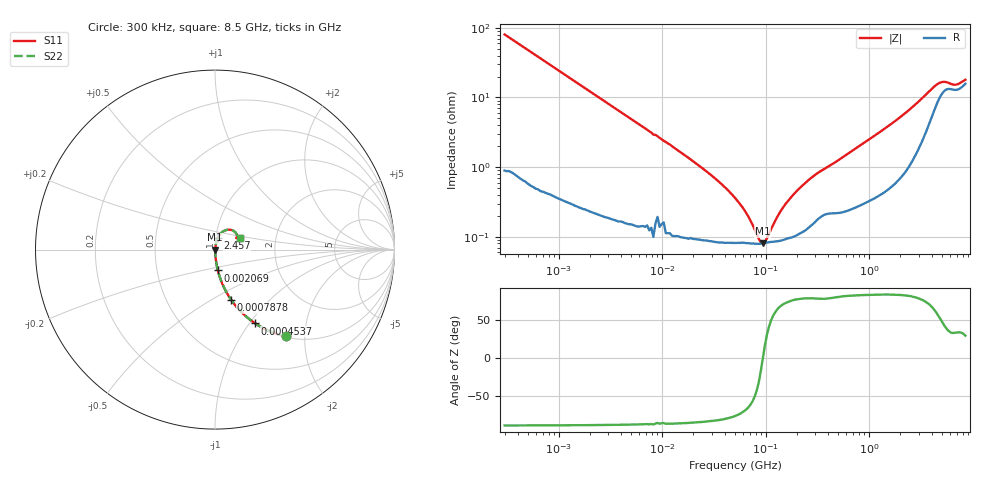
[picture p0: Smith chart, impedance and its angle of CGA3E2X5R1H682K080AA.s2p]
! S-parameter Generated by TDK Corporation
! Copyright(C) 2015 TDK Corporation.
! All Rights Reserved.
! TDK P/N: CGA3E2X5R1H682K080AA (Multilayer Ceramic Chip Capacitors)
! Property: C=6.8nF
! Size(LxWxT): 1.6x0.8x0.8mm, 0.063x0.031x0.031inches
! Model Type: s2p (Touchstone File Format Version 1.0)
! Frequency: DC=Yes Start=0.3MHz Stop=8500MHz 225points Log-sweep
! Note:
! Model Generated on Jun. 23, 2015
! Hash(MD5):
! Port Assignments:
!  1 ---| |--- 2
! Applicable Conditions:
!  Temperature = 25 degC
!  DC Bias Voltage = 0 V
!  Small Signal Operation
! Terms and conditions regarding TDK Simulation Models
! (1)This simulation model is being provided solely for informational purposes. Please refer to the specifications of the products in terms of detailed characteristics of such products.
! (2)In no event shall TDK Corporation of any of its subsidiaries be liable for any loss or damage arising, directly or indirectly,
!  From any information contained in this simulation model, including, but not limited to loss or damages arising from any inaccuracies, omissions or errors in connection with such information.
! (3)Any and all copyrights on this simulation model are owned by TDK Corporation.
!  Duplication or redistribution of this simulation model without prior written permission from TDK Corporation is prohibited.
! (4)This simulation model is subject to any modification or change without any prior notice.
! (5)Neither TDK Corporation nor any of its subsidiaries shall make any warranty, express or implied,
!  Including but not limited to the correctness, implied warranties of merchantability and fitness for a particular purpose with respect to this simulation models.
! (6)The use of this simulation model shall be deemed to have consented to the terms and conditions hereof.
# MHz S MA R 50
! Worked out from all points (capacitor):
!   224 points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, 300 kHz to 8.5 GHz, reference 50 ohm
!   read as one part in series: C = 6.59 nF near 314.1 kHz
!   lowest |Z| = 80.3 mohm at 93.93 MHz (marker M1)
!   series resonance near 94.01 MHz, so ESL is about 440 pH
!   S11 on the Smith chart (normalised r, x): 300 kHz: 1.02, -1.61; 453.7 kHz: 1.01, -1.07; 787.8 kHz: 1.01, -0.62; 2.069 MHz: 1.00, -0.24; 2.457 GHz: 1.02, +0.13; 8.5 GHz: 1.32, +0.17
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0.3  0.6229 -50.8  0.7754 38.5  0.7754 38.5  0.6229 -50.8
0.4537435  0.4683 -61.4  0.8779 27.9  0.8779 27.9  0.4683 -61.4
0.7877636  0.2936 -72.2  0.952 17.1  0.952 17.1  0.2936 -72.2
1.72111  0.1402 -80.9  0.9877 8.1  0.9877 8.1  0.1402 -80.9
2.068572  0.1172 -82.2  0.9909 6.7  0.9909 6.7  0.1172 -82.2
9.430415  0.02626 -85.5  0.9983 1.5  0.9983 1.5  0.02626 -85.5
28.42509  0.008075 -83.4  0.9991 0.5  0.9991 0.5  0.008075 -83.4
51.67171  0.00347 -76.3  0.9992 0.2  0.9992 0.2  0.00347 -76.3
65.02496  0.002179 -68.1  0.9992 0.1  0.9992 0.1  0.002179 -68.1
85.6787  0.0009325 -32.4  0.9992 0.0  0.9992 0.0  0.0009325 -32.4
93.92989  0.0008021 -0.3  0.9992 0.0  0.9992 0.0  0.0008021 -0.3
98.34885  0.0008463 16.5  0.9992 -0.0  0.9992 -0.0  0.0008463 16.5
129.5872  0.001934 63.6  0.9991 -0.1  0.9991 -0.1  0.001934 63.6
155.7485  0.002961 71.7  0.9991 -0.2  0.9991 -0.2  0.002961 71.7
205.2186  0.004729 76.6  0.9989 -0.3  0.9989 -0.3  0.004729 76.6
283.1228  0.007225 77.6  0.9985 -0.4  0.9985 -0.4  0.007225 77.6
1551.304  0.03926 80.7  0.9944 -2.2  0.9944 -2.2  0.03926 80.7
2456.696  0.06636 77.2  0.9875 -3.8  0.9875 -3.8  0.06636 77.2
4675.929  0.1449 47.9  0.9093 -6.8  0.9093 -6.8  0.1449 47.9
5367.404  0.1482 35.7  0.8839 -5.6  0.8839 -5.6  0.1482 35.7
6754.475  0.1346 28.4  0.884 -4.2  0.884 -4.2  0.1346 28.4
8500  0.155 24.6  0.8615 -4.3  0.8615 -4.3  0.155 24.6
